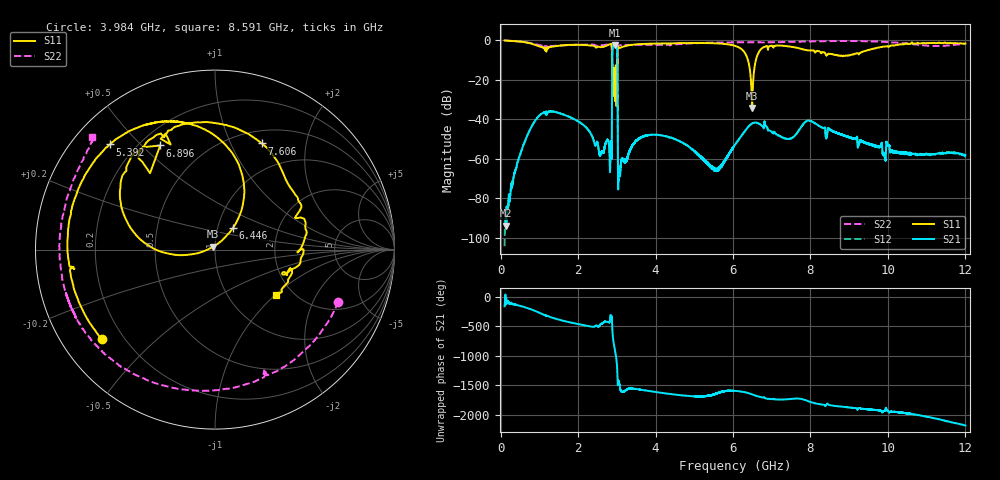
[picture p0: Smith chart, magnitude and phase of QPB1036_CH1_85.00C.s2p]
! TDS: K:\Engsetup\Winsaw\QPB1036_ALL
! Channel 1
! Ports=1 2
! seg 1=100.000000 1100.000000 101
! seg 2=1101.000000 1501.000000 401
! seg 3=1502.000000 2502.000000 101
! seg 4=2503.000000 3803.000000 1301
! seg 5=3804.000000 5004.000000 121
! seg 6=5005.000000 6005.000000 1001
! seg 7=6006.000000 8406.000000 241
! seg 8=8407.000000 10607.000000 2201
! seg 9=10608.000000 12008.000000 141
! Points=5609
! FailCode=0
! Topology=ALL_SE(12)
!VNA Cal loaded =QPB1036_ALL_85C
!PS1(V)= 5.000
!PS(mA)= 0.400
!PS2(V)= 0.630
!PS(mA)= -0.100
!PS3(V)= 0.630
!PS(mA)= 0.100
!PS4(V)= 1.170
!PS(mA)= -0.100
!Temp (C)= 85.00
# MHz S DB R 50
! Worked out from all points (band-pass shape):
!   5609 points, 100 MHz to 12.01 GHz, reference 50 ohm
!   highest |S21| = -2.63 dB at 2.947 GHz (marker M1); lowest = -93.7 dB at 140 MHz (marker M2)
!   |S21| within 3 dB of the highest: 2.886 GHz to 3.012 GHz (126.3 MHz wide, 4.28 % of centre)
!   lowest |S11| = -34.3 dB at 6.496 GHz (marker M3), VSWR 1.04, Z = 48.9 + j1.53 ohm
!   |S11| at or under -10 dB: 2.875878 GHz to 2.878608 GHz (2.729 MHz wide, 0.0949 % of centre); 2.883 GHz to 3.013 GHz (130.7 MHz wide, 4.43 % of centre); 6.385 GHz to 6.596 GHz (210.5 MHz wide, 3.24 % of centre)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
!   |S22| runs from -29.3 to -0.3 dB; largest |S21 - S12| = 0.0092
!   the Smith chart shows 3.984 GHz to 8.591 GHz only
!   S11 on the Smith chart (normalised r, x): 3.984 GHz: 0.12, -0.34; 5.392 GHz: 0.11, +0.41; 6.446 GHz: 1.18, +0.29; 6.896 GHz: 0.28, +0.57; 7.606 GHz: 0.65, +1.32; 8.591 GHz: 1.65, -1.01
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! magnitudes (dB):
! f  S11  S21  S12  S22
! 100 MHz  -0.3  -87.5  -104.1  -0.3
! 140 MHz  -0.4  -93.7  -88.0  -0.4
! 1.121 GHz  -4.1  -36.9  -36.9  -3.4
! 2.092 GHz  -2.5  -42.3  -42.3  -2.5
! 2.841 GHz  -2.1  -53.6  -53.6  -2.1
! 2.902 GHz  -15.9  -3.5  -3.4  -15.5
! 2.947 GHz  -25.8  -2.6  -2.6  -26.4
! 2.995 GHz  -23.6  -3.4  -3.4  -26.3
! 3.057 GHz  -4.1  -65.1  -64.0  -2.8
! 3.495 GHz  -2.3  -50.9  -51.0  -2.5
! 3.984 GHz  -1.9  -47.9  -47.8  -2.5
! 4.074 GHz  -1.8  -48.0  -48.0  -2.5
! 5.392 GHz  -1.6  -62.6  -63.1  -1.4
! 6.056 GHz  -3.0  -52.8  -53.1  -1.3
! 6.446 GHz  -16.1  -42.9  -42.9  -1.2
! 6.496 GHz  -34.3  -42.1  -42.1  -1.2
! 6.896 GHz  -3.7  -44.7  -44.7  -1.2
! 7.606 GHz  -3.8  -48.2  -48.2  -1.0
! 8.046 GHz  -5.4  -41.2  -41.2  -0.8
! 8.591 GHz  -7.5  -46.2  -46.2  -0.6
! 10.02 GHz  -3.6  -53.3  -53.3  -1.1
! 12.01 GHz  -1.9  -58.1  -58.4  -2.0
